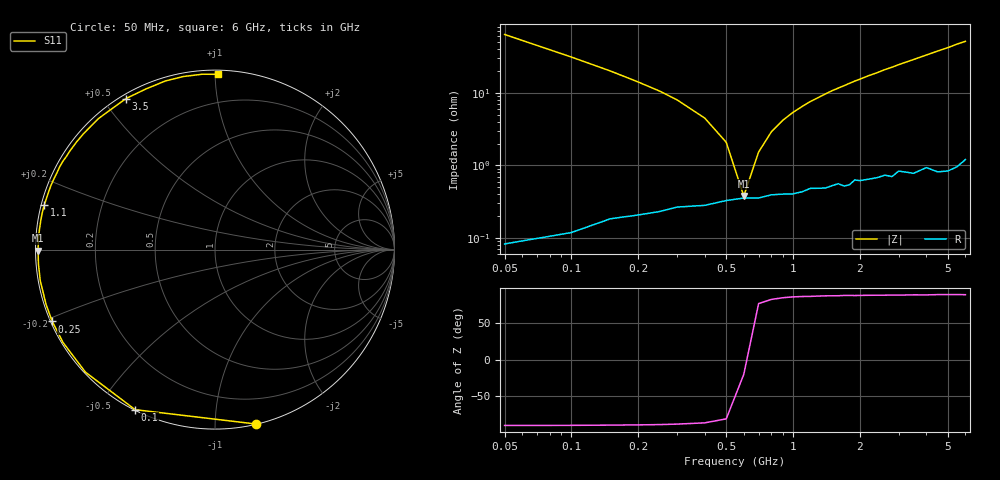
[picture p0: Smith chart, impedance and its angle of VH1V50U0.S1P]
! Infineon Technologies  Discrete & RF Semiconductors
! BB 814
! Si Tuning Diode in SOT23
! VR = 1.5 V
! S-Parameters:  July  1999
# GHz  S  MA  R  50
!  f  S11
! GHz  MAG  ANG
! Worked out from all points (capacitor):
!   34 points, 50 MHz to 6 GHz, reference 50 ohm
!   read as one part to ground: C = 50 pF near 50 MHz
!   lowest |Z| = 380 mohm at 600 MHz (marker M1)
!   series resonance near 608.1 MHz, so ESL is about 1.4 nH
!   S11 on the Smith chart (normalised r, x): 50 MHz: 0.00, -1.26; 100 MHz: 0.00, -0.62; 250 MHz: 0.00, -0.21; 1.1 GHz: 0.01, +0.13; 3.5 GHz: 0.02, +0.57; 6 GHz: 0.02, +1.02
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0.05  0.9987 -76.7
0.1  0.9966 -116.5
0.15  0.9937 -136.6
0.2  0.9923 -148.6
0.25  0.9912 -156.2
0.3  0.9896 -161.9
0.4  0.9889 -169.8
0.5  0.987 -175.3
0.6  0.9859 -179.7
0.7  0.9859 176.6
0.8  0.9844 173.4
1  0.9841 167.8
1.1  0.9831 165.3
1.4  0.9813 158.3
1.6  0.9789 154.0
1.7  0.9806 152.0
1.9  0.9769 147.8
2.2  0.9771 142.1
2.4  0.9765 138.7
2.6  0.9752 134.9
2.8  0.9769 131.7
3  0.9733 128.2
3.5  0.9768 120.5
4  0.9743 113.2
4.5  0.9793 106.4
5  0.9804 100.4
5.5  0.9797 94.1
6  0.9767 89.0
